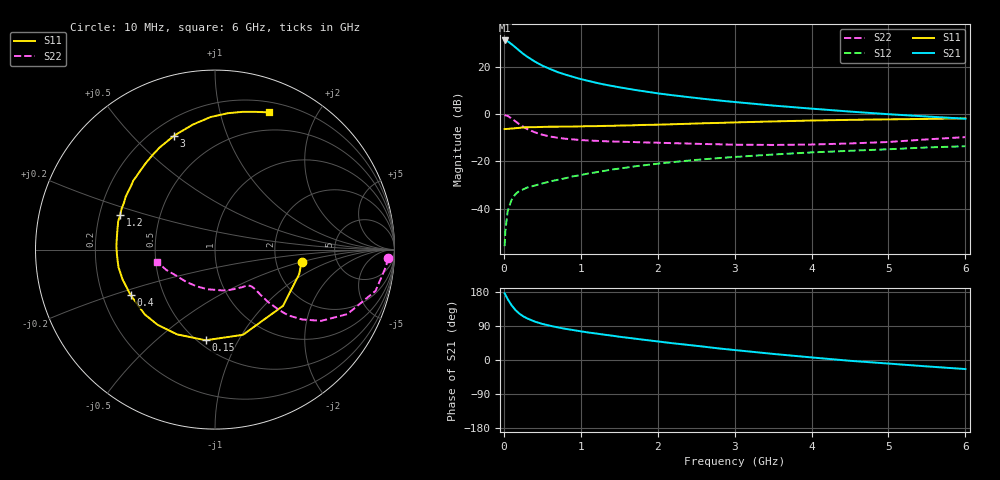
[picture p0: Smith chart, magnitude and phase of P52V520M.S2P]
! SIEMENS Small Signal Semiconductors
! BFP183
! Si NPN RF Bipolar Junction Transistor in SOT143
! VCE = 2.5 V  IC = 20 mA
! Common Emitter S-Parameters:  March  1996
# GHz  S  MA  R  50
!  f  S11  S21  S12  S22
! GHz  MAG  ANG  MAG  ANG  MAG  ANG  MAG  ANG
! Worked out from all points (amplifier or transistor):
!   36 points, 10 MHz to 6 GHz, reference 50 ohm
!   highest |S21| = 31.3 dB at 10 MHz (marker M1)
!   |S21| within 3 dB of that: start of sweep to 153.7 MHz
!   unconditionally stable (mu >= 1): 767.3 MHz to 5.509 GHz
!   at 250 MHz: K = 0.50, MSG = 28.8 dB, |S12| = -31.9 dB
!   at 1.4 GHz: K = 1.15, MAG = 15.4 dB, |S12| = -23.5 dB
!   at 6 GHz: K = 0.95, MSG = 5.8 dB, |S12| = -13.5 dB
!   S11 on the Smith chart (normalised r, x): 10 MHz: 2.80, -0.50; 150 MHz: 0.54, -0.74; 400 MHz: 0.32, -0.23; 1.2 GHz: 0.29, +0.16; 3 GHz: 0.29, +0.66; 6 GHz: 0.30, +1.42
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0.01  0.4877 -8.0  36.9 176.0  0.0016 79.1  0.9662 -2.8
0.02  0.4884 -16.4  36.78 172.4  0.0034 78.0  0.9565 -5.8
0.05  0.4918 -39.6  35.38 160.7  0.0089 76.9  0.9238 -14.4
0.1  0.4997 -71.8  30.86 144.6  0.0153 64.1  0.8201 -26.0
0.15  0.5078 -95.9  26.43 132.0  0.0203 56.7  0.712 -33.9
0.2  0.5175 -114.1  22.55 122.6  0.0236 52.2  0.6208 -38.8
0.25  0.5271 -127.4  19.3 115.5  0.0255 50.1  0.5488 -41.9
0.3  0.5325 -137.3  16.86 110.1  0.0279 49.5  0.4914 -43.3
0.4  0.5342 -151.7  13.25 101.5  0.0308 48.7  0.4167 -44.6
0.5  0.5411 -162.1  10.79 95.3  0.0342 48.4  0.3699 -44.8
0.6  0.5467 -169.8  9.179 90.4  0.0378 50.2  0.339 -44.7
0.7  0.547 -176.7  7.862 86.1  0.0408 51.2  0.3183 -44.6
0.9  0.5507 173.5  6.223 79.1  0.0484 52.3  0.2939 -45.0
1.1  0.562 163.6  5.112 72.5  0.0558 53.3  0.2786 -46.3
1.2  0.5623 159.8  4.68 69.9  0.0591 53.1  0.2741 -47.2
1.7  0.5863 143.1  3.301 56.5  0.0789 52.1  0.2581 -54.4
2.2  0.6169 128.8  2.535 44.1  0.0972 48.9  0.2445 -64.1
3  0.6743 109.8  1.827 26.3  0.1248 42.2  0.2269 -84.8
3.5  0.7077 100.0  1.536 16.1  0.1407 37.9  0.2245 -100.0
4.5  0.7636 84.5  1.145 -2.1  0.1687 28.9  0.2415 -132.4
5.5  0.8 73.6  0.9 -16.9  0.1986 21.1  0.2944 -157.4
6  0.821 68.7  0.808 -23.9  0.2108 16.4  0.329 -168.2
